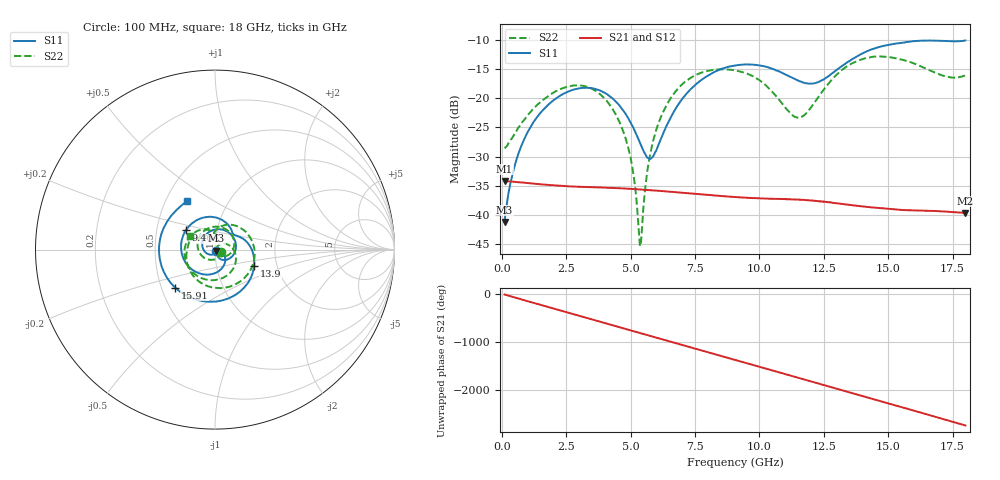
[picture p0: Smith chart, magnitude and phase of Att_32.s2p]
#  HZ  S  DB  R  50.00
! Rohde & Schwarz Vector Network Analyzer
! Rohde-Schwarz,ZNB40-4Port,1311601084101679,3.45
! Created: UTC 4/25/2025, 8:46:51 AM
! freq[Hz]  db:S11  ang:S11  db:S21  ang:S21  db:S12  ang:S12  db:S22  ang:S22
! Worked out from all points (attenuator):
!   1750 points, 100 MHz to 18 GHz, reference 50 ohm
!   highest |S21| = -34.18 dB at 100 MHz (marker M1); lowest = -39.7 dB at 18 GHz (marker M2)
!   lowest |S11| = -41.2 dB at 100 MHz (marker M3), VSWR 1.02, Z = 50.6 - j0.599 ohm
!   |S11| at or under -10 dB: start of sweep to end of sweep
!   |S22| runs from -45.3 to -12.8 dB; largest |S21 - S12| = 0.00013
!   S11 on the Smith chart (normalised r, x): 100 MHz: 1.01, -0.01; 9.464 GHz: 0.71, +0.16; 13.9 GHz: 1.52, -0.29; 15.91 GHz: 0.59, -0.28; 18 GHz: 0.64, +0.38
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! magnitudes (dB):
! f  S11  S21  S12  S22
! 100 MHz  -41.2  -34.2  -34.2  -28.6
! 540.1 MHz  -30.8  -34.3  -34.3  -25.8
! 1.144 GHz  -24.6  -34.6  -34.6  -22.2
! 2.055 GHz  -20.2  -34.9  -34.9  -18.9
! 3.088 GHz  -18.2  -35.2  -35.2  -17.8
! 3.979 GHz  -19.0  -35.3  -35.3  -20.0
! 4.654 GHz  -21.8  -35.4  -35.4  -25.1
! 5.053 GHz  -24.6  -35.5  -35.6  -31.6
! 5.371 GHz  -27.8  -35.6  -35.6  -45.3
! 5.688 GHz  -30.3  -35.7  -35.7  -31.2
! 6.067 GHz  -28.1  -35.9  -35.9  -24.4
! 6.568 GHz  -23.2  -36.0  -36.0  -19.9
! 7.223 GHz  -19.0  -36.3  -36.3  -16.8
! 9.055 GHz  -14.4  -36.9  -36.9  -15.2
! 9.464 GHz  -14.2  -37.0  -37.0  -15.7
! 11.38 GHz  -16.7  -37.4  -37.3  -23.2
! 12.04 GHz  -17.5  -37.6  -37.5  -21.3
! 12.99 GHz  -15.2  -38.0  -38.0  -16.0
! 13.9 GHz  -12.6  -38.5  -38.5  -13.4
! 15.02 GHz  -10.8  -38.9  -39.0  -12.9
! 15.91 GHz  -10.3  -39.2  -39.2  -13.9
! 18 GHz  -10.1  -39.7  -39.7  -16.1
